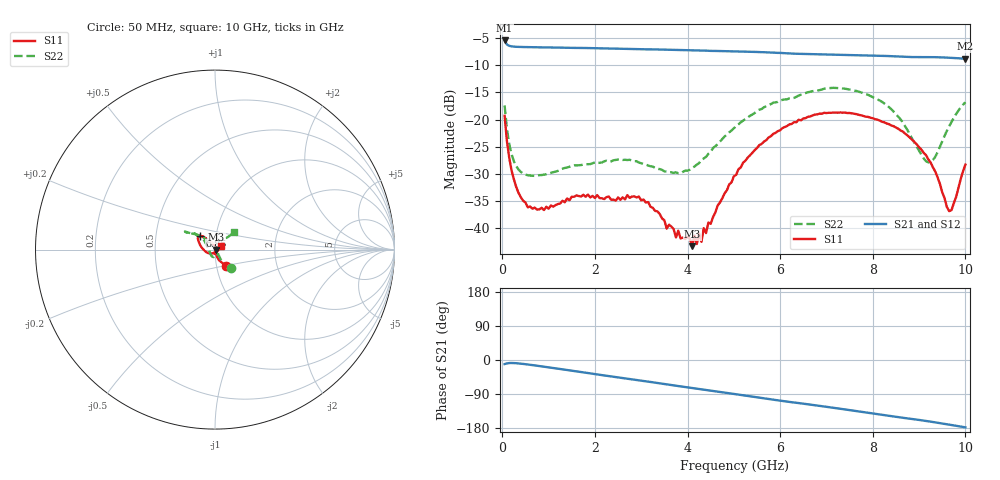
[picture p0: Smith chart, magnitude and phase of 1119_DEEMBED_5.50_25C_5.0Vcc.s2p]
!Hittite Microwave Corp.
!Digital Attenuator/PhaseShifter Rev 1.4.0
!Filename: C:\DATA\DATA\1119_DEEMBED_5.50_25C_5.0Vcc.s2p
!VNA ID: Agilent Technologies,N5224A,MY51441122,A.10.45.03
!Device type:
!2 Port Calibration.
!Temp(C): 25
!Lot Number:
!Serial Number:
!Operator:
!Misc:
!Attenuator:  5.500
# GHZ S DB R 50.0
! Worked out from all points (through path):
!   200 points, 50 MHz to 10 GHz, reference 50 ohm
!   highest |S21| = -5.43 dB at 50 MHz (marker M1); lowest = -8.8 dB at 10 GHz (marker M2)
!   group delay of S21, straight-line fit = 48.1 ps
!   lowest |S11| = -43.3 dB at 4.1 GHz (marker M3), VSWR 1.01, Z = 50.7 + j0.0433 ohm
!   |S11| at or under -10 dB: start of sweep to end of sweep
!   |S22| runs from -30.4 to -14.2 dB; largest |S21 - S12| = 0.0012
!   S11 on the Smith chart (normalised r, x): 50 MHz: 1.11, -0.20; 6.85 GHz: 0.84, +0.13; 10 GHz: 1.07, +0.04
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0.05  -19.31 -56.9  -5.43 -10.8  -5.43 -10.8  -17.40 -48.1
0.1  -24.00 -69.1  -6.19 -9.0  -6.18 -9.0  -21.71 -57.9
0.2  -29.39 -75.8  -6.52 -7.9  -6.52 -7.9  -26.40 -58.8
0.55  -36.17 -79.3  -6.66 -11.8  -6.66 -11.8  -30.27 -53.8
1.75  -33.86 -101.5  -6.82 -32.6  -6.82 -32.6  -28.25 -80.0
2.95  -34.19 -88.2  -7.04 -53.5  -7.05 -53.6  -27.93 -119.2
3.4  -37.41 -79.4  -7.09 -61.5  -7.09 -61.6  -29.13 -136.7
3.55  -40.10 -65.2  -7.11 -64.4  -7.12 -64.4  -29.62 -142.8
4.1  -43.33 3.6  -7.25 -74.0  -7.25 -74.1  -28.91 178.7
4.15  -41.36 2.0  -7.26 -74.9  -7.27 -74.9  -28.65 174.6
4.3  -42.53 33.5  -7.30 -77.4  -7.32 -77.5  -27.44 164.2
4.35  -40.00 39.1  -7.31 -78.2  -7.33 -78.3  -27.18 160.4
4.4  -40.92 44.2  -7.31 -79.2  -7.33 -79.3  -26.87 158.5
5.05  -30.18 104.7  -7.44 -90.4  -7.46 -90.5  -21.23 139.2
5.75  -23.31 126.1  -7.64 -102.9  -7.65 -102.9  -17.32 141.4
6.7  -19.26 136.1  -7.94 -118.6  -7.95 -118.6  -14.77 147.8
6.85  -18.91 137.1  -7.99 -121.1  -8.00 -121.1  -14.59 148.7
7.65  -19.01 148.1  -8.13 -134.7  -8.14 -134.8  -14.74 148.6
8.35  -20.85 160.2  -8.31 -147.2  -8.31 -147.2  -17.71 139.9
9.2  -27.34 -153.6  -8.49 -161.8  -8.51 -161.8  -27.89 104.1
9.65  -36.88 -63.6  -8.61 -170.6  -8.62 -170.6  -21.24 46.6
10  -28.30 30.6  -8.81 -177.8  -8.81 -177.8  -16.82 42.1
